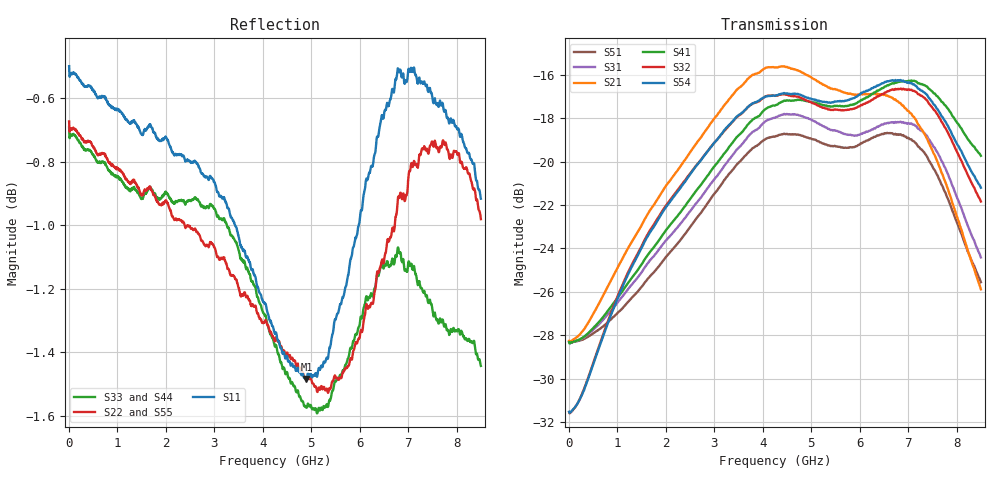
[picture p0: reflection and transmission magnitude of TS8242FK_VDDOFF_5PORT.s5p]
! Created with skrf (http://scikit-rf.org).
# Hz S RI R 50.0
!freq ReS11 ImS11 ReS12 ImS12 ReS13 ImS13
! ReS14 ImS14 ReS15 ImS15
! ReS21 ImS21 ReS22 ImS22 ReS23 ImS23
! ReS24 ImS24 ReS25 ImS25
! ReS31 ImS31 ReS32 ImS32 ReS33 ImS33
! ReS34 ImS34 ReS35 ImS35
! ReS41 ImS41 ReS42 ImS42 ReS43 ImS43
! ReS44 ImS44 ReS45 ImS45
! ReS51 ImS51 ReS52 ImS52 ReS53 ImS53
! ReS54 ImS54 ReS55 ImS55
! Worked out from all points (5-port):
!   1601 points, 10 MHz to 8.5 GHz, reference 50 ohm
!   strongest paths, dB at 10 MHz, 2.132 GHz, 4.255 GHz, 6.378 GHz, 8.5 GHz:
!     S54: -31.5, -21.7, -17.0, -16.5, -21.2
!     S32: -31.5, -21.7, -17.0, -17.0, -21.8
!     S41: -28.3, -22.8, -17.4, -16.7, -19.7
!     S21: -28.3, -20.8, -15.7, -16.9, -25.9
!     S31: -28.3, -23.3, -18.0, -18.4, -24.4
!     S51: -28.3, -24.1, -18.8, -18.8, -25.6
!   lowest |S11| = -1.5 dB at 4.902 GHz (marker M1), VSWR 11.74, Z = 21.3 + j98.1 ohm
!   |S11| at or under -10 dB: nowhere
